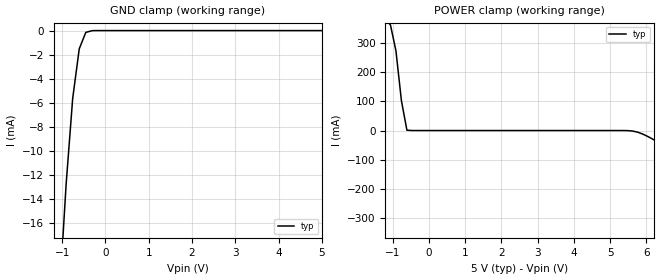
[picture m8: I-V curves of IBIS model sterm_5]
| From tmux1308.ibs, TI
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| sterm_5
[Model]   sterm_5
Model_type   Terminator
|   typ   min   max
C_comp   1.008417e-12   NA   NA
[Voltage Range]   5   NA   NA
[Temperature Range]   27   NA   NA
[Power Clamp Reference]   5   NA   NA
[GND Clamp Reference]   0   NA   NA
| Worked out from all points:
|   GND clamp passes 1 mA (typ) near -0.55 V on its own axis
|   POWER clamp passes 1 mA (typ) near -0.60 V on its own axis
[GND Clamp]
|   Voltage   I(typ)   I(min)   I(max)
-10V      -75.72kA   NA         NA
-1.061V   -21.84mA   NA         NA
-909.1mV  -12.79mA   NA         NA
-757.6mV  -5.651mA   NA         NA
-606.1mV  -1.521mA   NA         NA
-454.5mV  -150.8uA   NA         NA
-303mV    -3.403uA   NA         NA
5V        2.454nA    NA         NA
[POWER Clamp]
|   Voltage   I(typ)   I(min)   I(max)
-5V       1.511A     NA         NA
-1.061V   360.5mA    NA         NA
-909.1mV  272.3mA    NA         NA
-757.6mV  101.9mA    NA         NA
-606.1mV  1.02mA     NA         NA
5.455V    -150.8uA   NA         NA
5.758V    -5.651mA   NA         NA
6.061V    -21.84mA   NA         NA
6.515V    -55.15mA   NA         NA
7.879V    -173.7mA   NA         NA
8.03V     -406.8mA   NA         NA
10V       -20.06kA   NA         NA
